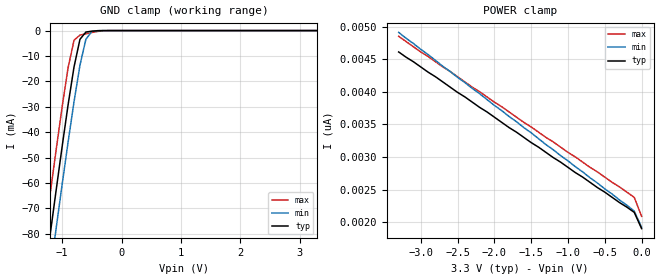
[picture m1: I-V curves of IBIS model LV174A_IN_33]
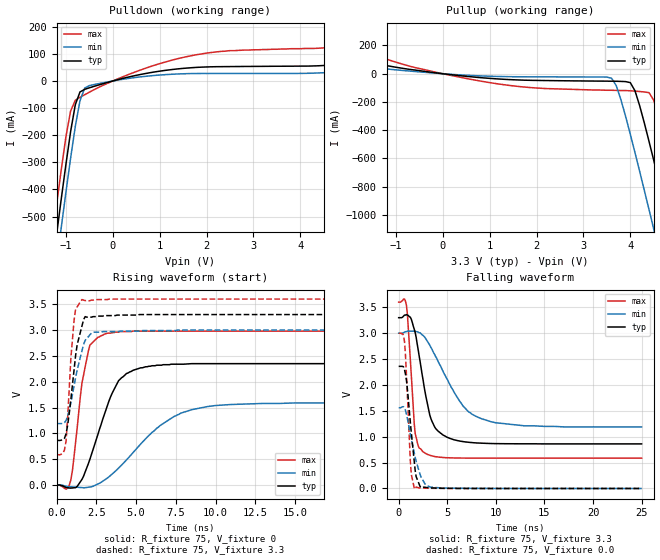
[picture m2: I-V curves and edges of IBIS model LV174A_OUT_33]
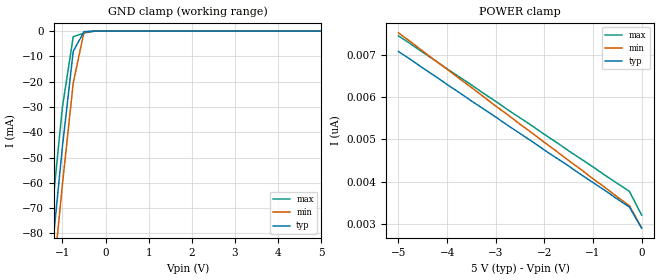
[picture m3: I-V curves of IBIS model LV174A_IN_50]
| TEXAS INSTRUMENTS INCORPORATED
| Standard Linear and Logic Group
| IBIS Model of SN74LV174A
| HEX D-TYPE FLIP-FLOP WITH CLEAR
| SOIC 16-pin (D), SOP 16-pin (NS), SSOP 16-pin (DB), TSSOP 16-pin (PW)
| and TVSOP 16-pin (DGV) Package
[IBIS Ver]   3.2
[Comment Char]  |_char
[File Name]   lv174a.ibs
[File Rev]   2.0 H_die
[Date]   May 24, 2000
[Source]   Data created from HSPICE simulations at TI-SLL.
[Notes]   The following is an IBIS list for the LV174A.
|   Please contact sllibis@ti.com with questions and
|   comments concerning SLL IBIS models.
[Disclaimer] Property of Texas Instruments Incorporated.  Unauthorized
   reproduction and/or distribution is strictly prohibited.
   This product is protected under copyright law.
   Created 2000, (C) Copyright 2000, Texas Instruments Inc.,
   All Rights Reserved.
   UNLESS THERE IS A SIGNED, WRITTEN AGREEMENT TO THE
   CONTRARY, TEXAS INSTRUMENTS () IS PROVIDING THE IBIS
   MODELS  AND WITHOUT ANY WARRANTY, EXPRESSED OR
   IMPLIED.  TI assumes no liability for:
   1) the accuracy of the IBIS models provided to your
   company;
   2) the proper functioning of these IBIS Models in your
   design or for any resulting applications; or
   3) infringement of patents, copyrights or intellectual
   property rights resulting from your use of these IBIS
   models.
   TI provides IBIS Models as a service to our customers.
   You and your company shall not distribute, sell or give
   these models to anyone else without prior written
   permission from TI.
   TI reserves the right to make changes to our products or
   to discontinue any semiconductor product or service
   without notice, and advises our customers to obtain the
   latest version of relevant information to verify, before
   placing orders, that the information being relied on is
   current.
   Please be aware that your receipt and use of the IBIS
   information provided shall serve as acceptance of these
   terms and conditions.  If you do not accept these terms,
   you should return or destroy the IBIS models and any
   other accompanying information immediately.
|   Component LV174A_D
[Component]   LV174A_D
[Manufacturer]  Texas Instruments, Inc.
[Package]
|   typ   min   max
R_pkg   0.039   0.028   0.049
L_pkg   3.453nH   2.350nH   4.375nH
C_pkg   0.521pF   0.254pF   0.708pF
[Pin]   signal_name   model_name   R_pin   L_pin   C_pin
1   CLR_NOT   LV174A_IN   0.042   4.336nH   0.703pF
2   1Q   LV174A_OUT   0.049   3.778nH   0.634pF
3   1D   LV174A_IN   0.028   3.449nH   0.518pF
4   2D   LV174A_IN   0.029   2.393nH   0.254pF
5   2Q   LV174A_OUT   0.028   2.350nH   0.264pF
6   3D   LV174A_IN   0.048   3.312nH   0.483pF
7   3Q   LV174A_OUT   0.043   3.629nH   0.604pF
8   GND   GND   0.044   4.375nH   0.708pF
9   CLK   LV174A_IN   0.042   4.336nH   0.703pF
10   4Q   LV174A_OUT   0.049   3.778nH   0.634pF
11   4D   LV174A_IN   0.028   3.449nH   0.518pF
12   5Q   LV174A_OUT   0.029   2.393nH   0.255pF
13   5D   LV174A_IN   0.028   2.350nH   0.264pF
14   6D   LV174A_IN   0.048   3.312nH   0.483pF
15   6Q   LV174A_OUT   0.043   3.629nH   0.604pF
16   VCC   POWER   0.044   4.375nH   0.708pF
|   Component LV174A_NS
[Component]   LV174A_NS
[Manufacturer]  Texas Instruments, Inc.
[Package]
|   typ   min   max
R_pkg   0.042   0.035   0.049
L_pkg   3.147nH   2.164nH   4.219nH
C_pkg   0.404pF   0.241pF   0.562pF
[Pin]   signal_name   model_name   R_pin   L_pin   C_pin
1   CLR_NOT   LV174A_IN   0.049   4.215nH   0.562pF
2   1Q   LV174A_OUT   0.046   3.675nH   0.480pF
3   1D   LV174A_IN   0.037   2.527nH   0.332pF
4   2D   LV174A_IN   0.035   2.164nH   0.241pF
5   2Q   LV174A_OUT   0.035   2.164nH   0.241pF
6   3D   LV174A_IN   0.037   2.527nH   0.332pF
7   3Q   LV174A_OUT   0.046   3.675nH   0.480pF
8   GND   GND   0.049   4.215nH   0.562pF
9   CLK   LV174A_IN   0.049   4.219nH   0.562pF
10   4Q   LV174A_OUT   0.046   3.679nH   0.480pF
11   4D   LV174A_IN   0.037   2.531nH   0.333pF
12   5Q   LV174A_OUT   0.035   2.168nH   0.241pF
13   5D   LV174A_IN   0.035   2.168nH   0.241pF
14   6D   LV174A_IN   0.037   2.531nH   0.333pF
15   6Q   LV174A_OUT   0.046   3.679nH   0.480pF
16   VCC   POWER   0.049   4.219nH   0.562pF
|   Component LV174A_DB
[Component]   LV174A_DB
[Manufacturer]  Texas Instruments, Inc.
[Package]
|   typ   min   max
R_pkg   0.048   0.046   0.050
L_pkg   3.536nH   3.213nH   3.798nH
C_pkg   0.376pF   0.314pF   0.440pF
[Pin]   signal_name   model_name   R_pin   L_pin   C_pin
1   CLR_NOT   LV174A_IN   0.048   3.797nH   0.377pF
2   1Q   LV174A_OUT   0.046   3.723nH   0.440pF
3   1D   LV174A_IN   0.048   3.409nH   0.372pF
4   2D   LV174A_IN   0.049   3.213nH   0.314pF
5   2Q   LV174A_OUT   0.049   3.213nH   0.314pF
6   3D   LV174A_IN   0.048   3.409nH   0.372pF
7   3Q   LV174A_OUT   0.046   3.723nH   0.440pF
8   GND   GND   0.048   3.798nH   0.377pF
9   CLK   LV174A_IN   0.048   3.797nH   0.377pF
10   4Q   LV174A_OUT   0.046   3.725nH   0.440pF
11   4D   LV174A_IN   0.048   3.409nH   0.372pF
12   5Q   LV174A_OUT   0.049   3.214nH   0.314pF
13   5D   LV174A_IN   0.050   3.216nH   0.314pF
14   6D   LV174A_IN   0.048   3.409nH   0.372pF
15   6Q   LV174A_OUT   0.047   3.729nH   0.440pF
16   VCC   POWER   0.048   3.797nH   0.377pF
|   Component LV174A_PW
[Component]   LV174A_PW
[Manufacturer]  Texas Instruments, Inc.
[Package]
|   typ   min   max
R_pkg   0.045   0.038   0.051
L_pkg   2.593nH   2.447nH   3.080nH
C_pkg   0.281pF   0.243pF   0.377pF
[Pin]   signal_name   model_name   R_pin   L_pin   C_pin
1   CLR_NOT   LV174A_IN   0.040   3.080nH   0.377pF
2   1Q   LV174A_OUT   0.038   2.458nH   0.281pF
3   1D   LV174A_IN   0.051   2.512nH   0.255pF
4   2D   LV174A_IN   0.051   2.447nH   0.243pF
5   2Q   LV174A_OUT   0.051   2.447nH   0.243pF
6   3D   LV174A_IN   0.051   2.512nH   0.255pF
7   3Q   LV174A_OUT   0.038   2.458nH   0.281pF
8   GND   GND   0.040   3.080nH   0.377pF
9   CLK   LV174A_IN   0.039   2.832nH   0.316pF
10   4Q   LV174A_OUT   0.038   2.460nH   0.279pF
11   4D   LV174A_IN   0.051   2.512nH   0.255pF
12   5Q   LV174A_OUT   0.051   2.447nH   0.243pF
13   5D   LV174A_IN   0.051   2.447nH   0.243pF
14   6D   LV174A_IN   0.051   2.512nH   0.255pF
15   6Q   LV174A_OUT   0.038   2.459nH   0.279pF
16   VCC   POWER   0.039   2.832nH   0.316pF
|   Component LV174A_DGV
[Component]   LV174A_DGV
[Manufacturer]  Texas Instruments, Inc.
[Package]
|   typ   min   max
R_pkg   0.039   0.033   0.045
L_pkg   2.543nH   2.320nH   2.938nH
C_pkg   0.386pF   0.334pF   0.449pF
[Pin]   signal_name   model_name   R_pin   L_pin   C_pin
1   CLR_NOT   LV174A_IN   0.035   2.907nH   0.417pF
2   1Q   LV174A_OUT   0.042   2.558nH   0.446pF
3   1D   LV174A_IN   0.038   2.341nH   0.345pF
4   2D   LV174A_IN   0.038   2.320nH   0.334pF
5   2Q   LV174A_OUT   0.039   2.322nH   0.334pF
6   3D   LV174A_IN   0.038   2.353nH   0.342pF
7   3Q   LV174A_OUT   0.040   2.536nH   0.441pF
8   GND   GND   0.033   2.897nH   0.418pF
9   CLK   LV174A_IN   0.035   2.927nH   0.419pF
10   4Q   LV174A_OUT   0.045   2.632nH   0.449pF
11   4D   LV174A_IN   0.039   2.368nH   0.347pF
12   5Q   LV174A_OUT   0.039   2.330nH   0.335pF
13   5D   LV174A_IN   0.039   2.320nH   0.335pF
14   6D   LV174A_IN   0.039   2.361nH   0.345pF
15   6Q   LV174A_OUT   0.041   2.573nH   0.446pF
16   VCC   POWER   0.035   2.938nH   0.420pF
[Model Selector]   LV174A_IN
LV174A_IN_33   3.3-V Vcc Input Model
LV174A_IN_50   5.0-V Vcc Input Model
[Model Selector]   LV174A_OUT
LV174A_OUT_33   3.3-V Vcc Output Model
LV174A_OUT_50   5.0-V Vcc Output Model
| Models and submodels in the file (4): LV174A_IN_33 (Input), LV174A_OUT_33 (Output), LV174A_IN_50 (Input), LV174A_OUT_50 (Output)
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|   Model LV174A_IN_33
[Model]   LV174A_IN_33
Model_type  Input
Polarity   Inverting
Vinl = 0.99
Vinh = 2.31
| variable   typ   min   max
C_comp   1.35pf   1.01pf   1.69pf
[Temperature Range]   25   85   -40
[Voltage Range]   3.3   3.0   3.6
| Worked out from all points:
|   GND clamp passes 1 mA (typ) near -0.61 V on its own axis
[GND Clamp]
|   Voltage   I(typ)   I(min)   I(max)
-3.3V     -460mA     -475mA     -445mA
-1.3V     -97.5mA    -113mA     -81.5mA
-1.2V     -79.9mA    -95mA      -63.9mA
-1.1V     -62.6mA    -77.6mA    -46.7mA
-1V       -45.6mA    -60.5mA    -30mA
-900mV    -29.2mA    -43.9mA    -14.6mA
-800mV    -14.3mA    -28mA      -3.81mA
-700mV    -3.42mA    -13.6mA    -1.78mA
-600mV    -581uA     -3.4mA     -1.25mA
-500mV    -233uA     -353uA     -759uA
-400mV    -58.1uA    -21.9uA    -324uA
3.3V      1.9nA      2.34nA     1.69nA
[POWER Clamp]
|   Voltage   I(typ)   I(min)   I(max)
-3.3V     4.61nA     4.91nA     4.85nA
-3V       4.38nA     4.65nA     4.61nA
-100mV    2.15nA     2.17nA     2.38nA
0V        1.9nA      1.92nA     2.09nA
|   Model LV174A_OUT_33
[Model]   LV174A_OUT_33
Model_type  Output
Polarity   Non-Inverting
Vmeas = 1.65v
Cref = 15pf
| variable   typ   min   max
C_comp   5.60pf   4.20pf   7.00pf
[Temperature Range]   25   85   -40
[Voltage Range]   3.3   3.0   3.6
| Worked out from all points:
|   slope of the pulldown table from 0 to 0.495 V, typ, clamps not added: 24 ohm
|   slope of the pullup table from 0 to 0.495 V, typ, clamps not added: 27.2 ohm
|   rising waveform, R_fixture 75, V_fixture 0: 20-80 % time 1.6ns typ, 3.25ns min, 746ps max; typ from 0 V to 2.35 V
|   falling waveform, R_fixture 75, V_fixture 3.3: 20-80 % time 1.43ns typ, 3.29ns min, 610ps max; typ from 3.3 V to 0.862 V
|   rising waveform, R_fixture 75, V_fixture 3.3: 20-80 % time 595ps typ, 759ps min, 377ps max; typ from 0.862 V to 3.3 V
|   falling waveform, R_fixture 75, V_fixture 0.0: 20-80 % time 715ps typ, 1.13ns min, 436ps max; typ from 2.36 V to 0 V
[Pulldown]
|   Voltage   I(typ)   I(min)   I(max)
-3.3V     -3.5A      -3.6A      -3.4A
-1.3V     -703mA     -808mA     -592mA
-1.2V     -568mA     -673mA     -458mA
-1.1V     -436mA     -541mA     -328mA
-900mV    -187mA     -285mA     -111mA
-800mV    -87.9mA    -168mA     -71.2mA
-700mV    -40.4mA    -73.1mA    -60mA
-600mV    -30.8mA    -26.2mA    -50.7mA
-500mV    -25.2mA    -17mA      -41.3mA
1.7V      49.2mA     27.4mA     94.1mA
4.8V      61.3mA     33.4mA     127mA
6.6V      103mA      59.8mA     194mA
[Pullup]
|   Voltage   I(typ)   I(min)   I(max)
-3.3V     172mA      95.9mA     319mA
500mV     -18.4mA    -10.6mA    -33.4mA
3.6V      -52.9mA    -31.7mA    -117mA
3.8V      -54.3mA    -184mA     -119mA
4V        -63mA      -429mA     -121mA
4.1V      -121mA     -559mA     -123mA
4.4V      -480mA     -963mA     -134mA
4.5V      -613mA     -1.1A      -188mA
4.8V      -1.02A     -1.51A     -558mA
4.9V      -1.16A     -1.65A     -693mA
5.2V      -1.58A     -2.07A     -1.11A
6.6V      -3.55A     -4.04A     -3.07A
[Ramp]
| variable   typ   min   max
dV/dt_r   1.42E+00/1.58E-09   9.66E-01/3.29E-09   1.80E+00/6.90E-10
dV/dt_f   1.50E+00/1.42E-09   1.11E+00/3.31E-09   1.85E+00/5.70E-10
R_load = 75
[Rising Waveform]
R_fixture = 75
V_fixture = 0
|   Time   V(typ)   V(min)   V(max)
0s        0V         0V         0V
800ps     -56.8mV    -31.1mV    -2.26mV
1ns       -55.2mV    -35.5mV    285mV
1.6ns     111mV      -49mV      1.98V
2ns       414mV      -41.1mV    2.59V
3ns       1.36V      95.2mV     2.92V
4.4ns     2.16V      488mV      2.97V
6.5ns     2.32V      1.15V      2.98V
8.5ns     2.35V      1.46V      2.98V
25ns      2.35V      1.59V      2.98V
[Falling Waveform]
R_fixture = 75
V_fixture = 3.3
V_fixture_min = 3.0
V_fixture_max = 3.6
|   Time   V(typ)   V(min)   V(max)
0s        3.3V       3V         3.6V
800ps     3.36V      3.03V      3.54V
1.2ns     3.31V      3.04V      2.49V
1.7ns     3.01V      3.04V      1.06V
2.5ns     2.11V      2.96V      710mV
3.2ns     1.42V      2.77V      643mV
3.8ns     1.16V      2.55V      615mV
6.6ns     907mV      1.6V       588mV
8.5ns     876mV      1.35V      587mV
25ns      862mV      1.19V      586mV
[Rising Waveform]
R_fixture = 75
V_fixture = 3.3
V_fixture_min = 3.0
V_fixture_max = 3.6
|   Time   V(typ)   V(min)   V(max)
0s        862mV      1.19V      586mV
400ps     876mV      1.19V      617mV
600ps     994mV      1.25V      853mV
900ps     1.65V      1.59V      2.45V
1.1ns     2.22V      1.92V      3.18V
1.3ns     2.72V      2.23V      3.45V
1.6ns     3.08V      2.6V       3.59V
1.8ns     3.26V      2.8V       3.57V
2.3ns     3.26V      2.96V      3.58V
25ns      3.3V       3V         3.6V
[Falling Waveform]
R_fixture = 75
V_fixture = 0.0
|   Time   V(typ)   V(min)   V(max)
0s        2.36V      1.56V      3V
400ps     2.36V      1.58V      2.99V
600ps     2.3V       1.56V      2.84V
800ps     2.09V      1.44V      2.2V
1.2ns     1.28V      1.05V      529mV
1.3ns     1.08V      954mV      273mV
1.7ns     344mV      600mV      -13mV
2.3ns     18.2mV     224mV      11.2mV
3.3ns     11.2mV     25.8mV     4.11mV
25ns      0V         1.39uV     5.72uV
|   Model LV174A_IN_50
[Model]   LV174A_IN_50
Model_type  Input
Polarity   Inverting
Vinl = 1.5
Vinh = 3.5
| variable   typ   min   max
C_comp   1.35pf   1.01pf   1.69pf
[Temperature Range]   25   85   -40
[Voltage Range]   5.0   4.5   5.5
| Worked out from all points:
|   GND clamp passes 1 mA (typ) near -0.52 V on its own axis
[GND Clamp]
|   Voltage   I(typ)   I(min)   I(max)
-5V       -773mA     -786mA     -758mA
-1.5V     -133mA     -148mA     -117mA
-1.25V    -88.7mA    -104mA     -72.7mA
-1V       -45.6mA    -60.5mA    -30mA
-750mV    -7.99mA    -20.5mA    -2.23mA
-500mV    -233uA     -353uA     -759uA
-250mV    -2.63nA    -182nA     -26.9uA
5V        2.9nA      3.64nA     2.54nA
[POWER Clamp]
|   Voltage   I(typ)   I(min)   I(max)
-5V       7.08nA     7.52nA     7.45nA
-1.5V     4.37nA     4.5nA      4.73nA
-250mV    3.4nA      3.43nA     3.77nA
0V        2.9nA      2.91nA     3.21nA
